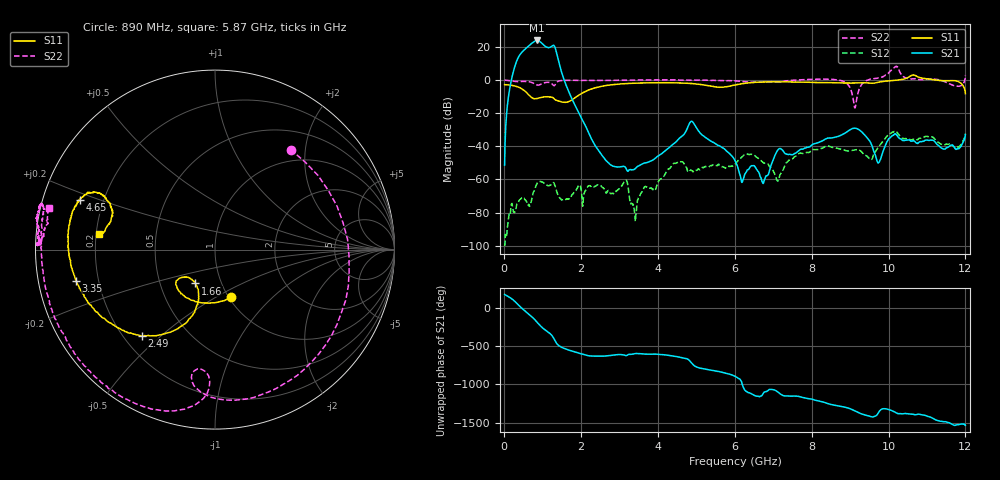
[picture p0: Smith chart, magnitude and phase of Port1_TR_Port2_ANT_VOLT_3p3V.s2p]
! Created Mon Aug 25 10:58:38 2025
# hz S ma R 50
! 2 Port Network Data from SP1.SP block
! freq  magS11  angS11  magS21  angS21  magS12  angS12  magS22  angS22
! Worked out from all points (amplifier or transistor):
!   1200 points, 10 MHz to 12 GHz, reference 50 ohm
!   highest |S21| = 23.8 dB at 860 MHz (marker M1)
!   |S21| within 3 dB of that: 652.4 MHz to 1.038 GHz (385.8 MHz wide, 45.6 % of centre)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
!   unconditionally stable (mu >= 1): start of sweep to 3.539 GHz; 4.511 GHz to 7.641 GHz; 8.675 GHz to 9.467 GHz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
!   at 2.01 GHz: K = 887.45, MAG = -10.2 dB, |S12| = -67.6 dB
!   at 6.01 GHz: K = 3036.08, MAG = -36.8 dB, |S12| = -50.9 dB
!   at 12 GHz: K = -794.77, MSG = -0.2 dB, |S12| = -32.5 dB
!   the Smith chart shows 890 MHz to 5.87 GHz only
!   S11 on the Smith chart (normalised r, x): 890 MHz: 1.03, -0.59; 1.66 GHz: 0.75, -0.30; 2.49 GHz: 0.27, -0.44; 3.35 GHz: 0.12, -0.11; 4.65 GHz: 0.11, +0.18; 5.87 GHz: 0.21, +0.06
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1e7  0.7209 178.6  0.002686 172.3  9.658e-06 -50.0  0.9837 176.3
3.5e8  0.6191 126.2  4.361 46.2  0.0001912 128.4  0.8933 2.2
5.2e8  0.4782 84.7  8.04 -33.5  0.000268 82.0  0.9059 -99.3
7.1e8  0.298 8.2  12.53 -114.3  0.000233 124.3  0.845 -178.9
8e8  0.2704 -35.0  14.87 -158.6  0.0005271 110.3  0.7546 128.1
8.6e8  0.2755 -60.8  15.53 168.1  0.0007751 88.1  0.7009 79.5
8.9e8  0.2818 -71.2  15.26 151.2  0.0008426 74.4  0.6986 52.9
1.01e9  0.3035 -102.4  11.8 91.8  0.0008127 29.4  0.7973 -31.5
1.22e9  0.3041 -132.4  10.04 8.9  0.0006963 -25.7  0.7987 -95.6
1.33e9  0.2528 -140.9  8.989 -79.6  0.0005968 -112.0  0.7366 -92.3
1.41e9  0.2343 -138.8  3.809 -130.0  0.0003146 -159.0  0.9152 -102.6
1.66e9  0.218 -120.0  0.4977 170.5  0.0002565 140.3  0.9737 -129.1
2.01e9  0.3882 -108.9  0.07008 117.7  0.0004149 59.6  0.9691 -151.7
2.49e9  0.6304 -130.2  0.006512 87.3  0.000672 57.3  0.9671 -174.9
3.35e9  0.7938 -167.4  0.001955 115.1  0.0001662 -5.1  0.9851 166.0
4.01e9  0.8231 172.8  0.005161 110.9  0.0008639 73.8  1.009 167.3
4.65e9  0.8035 159.8  0.02113 62.8  0.00331 -19.1  0.9853 174.4
5.87e9  0.6525 172.3  0.005903 -149.5  0.002441 -17.4  0.9544 166.1
6.01e9  0.7044 175.7  0.003606 -178.6  0.002858 -3.2  0.9358 159.1
8.01e9  0.8418 159.3  0.01107 -114.3  0.007721 -92.7  1.04 56.2
1.001e10  0.9377 127.7  0.01707 108.4  0.02299 129.5  1.661 137.3
1.2e10  0.3847 75.2  0.02251 -97.6  0.02364 -87.9  1.412 64.2
